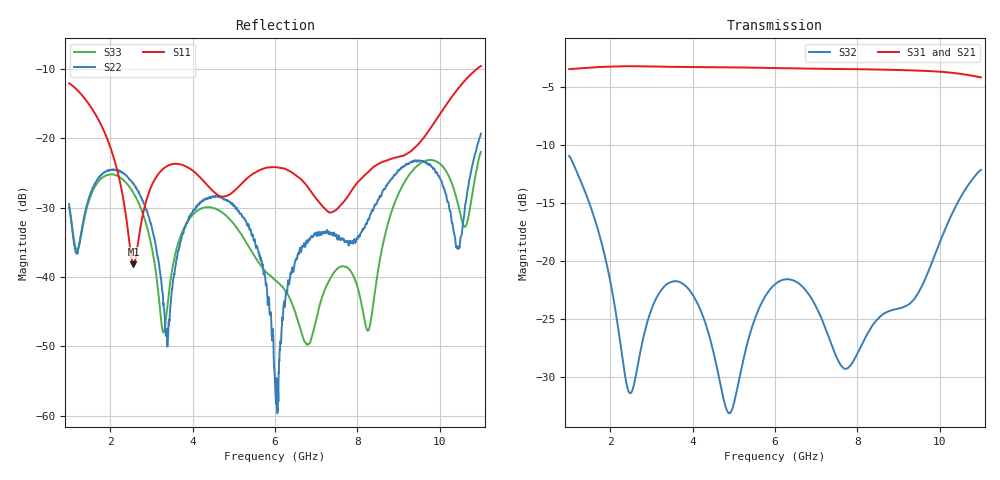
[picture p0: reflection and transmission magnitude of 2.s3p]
!The following data was pulled from an Agilent PNA
!This sNp file was generated from the data in the RF Test software
!NOTE:  Smoothing/Math/Corrections applied on any given trace ARE included in the data saved here
# MHz S dB R 50
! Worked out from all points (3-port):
!   1601 points, 1 GHz to 11 GHz, reference 50 ohm
!   strongest paths, dB at 1 GHz, 3.5 GHz, 6 GHz, 8.5 GHz, 11 GHz:
!     S31: -3.4, -3.2, -3.3, -3.5, -4.1
!     S21: -3.4, -3.2, -3.3, -3.5, -4.1
!     S32: -10.9, -21.8, -22.0, -25.0, -12.1
!   lowest |S11| = -38.1 dB at 2.562 GHz (marker M1), VSWR 1.03, Z = 49 + j0.739 ohm
!   |S11| at or under -10 dB: start of sweep to 10.9 GHz
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1000  -12.06 131.8  -3.42 -64.8  -3.42 -63.9
      -3.42 -63.9  -29.47 21.2  -10.92 -85.6
      -3.42 -63.9  -10.91 -85.6  -29.96 18.9
2562.5  -38.13 142.6  -3.17 -168.0  -3.17 -168.1
        -3.17 -168.0  -26.58 120.5  -30.82 -74.7
        -3.17 -168.1  -30.82 -74.7  -27.86 117.9
3375  -24.00 -170.9  -3.21 137.3  -3.22 137.2
      -3.21 137.3  -48.42 138.1  -21.98 -74.5
      -3.21 137.2  -21.97 -74.5  -44.76 -75.0
4175  -25.59 173.6  -3.25 83.3  -3.25 83.3
      -3.25 83.3  -29.32 173.4  -24.08 -114.4
      -3.25 83.3  -24.07 -114.4  -30.22 -170.9
5400  -25.37 -144.6  -3.29 -0.5  -3.29 -0.6
      -3.29 -0.5  -33.06 85.7  -26.18 -58.4
      -3.29 -0.6  -26.16 -58.4  -35.98 64.1
6000  -24.14 -152.0  -3.33 -42.0  -3.33 -42.1
      -3.32 -42.0  -55.23 79.2  -22.00 -83.9
      -3.32 -42.2  -21.98 -83.9  -40.42 -32.1
7937.5  -26.86 -96.0  -3.43 -178.8  -3.42 -179.0
        -3.43 -178.8  -34.91 118.7  -28.40 -103.4
        -3.42 -179.1  -28.40 -103.4  -40.30 1.6
9306.25  -21.82 -83.5  -3.52 81.0  -3.52 80.7
         -3.52 81.0  -23.44 71.3  -23.55 -102.7
         -3.52 80.7  -23.55 -102.6  -24.87 53.2
10437.5  -12.87 -85.5  -3.78 -4.8  -3.80 -5.2
         -3.77 -4.8  -35.77 -91.5  -14.92 -116.4
         -3.79 -5.3  -14.92 -116.4  -29.32 -56.1
11000  -9.57 -109.8  -4.10 -46.8  -4.13 -48.5
       -4.12 -47.9  -19.31 140.6  -12.11 -144.4
       -4.13 -48.6  -12.11 -144.4  -21.96 140.1
